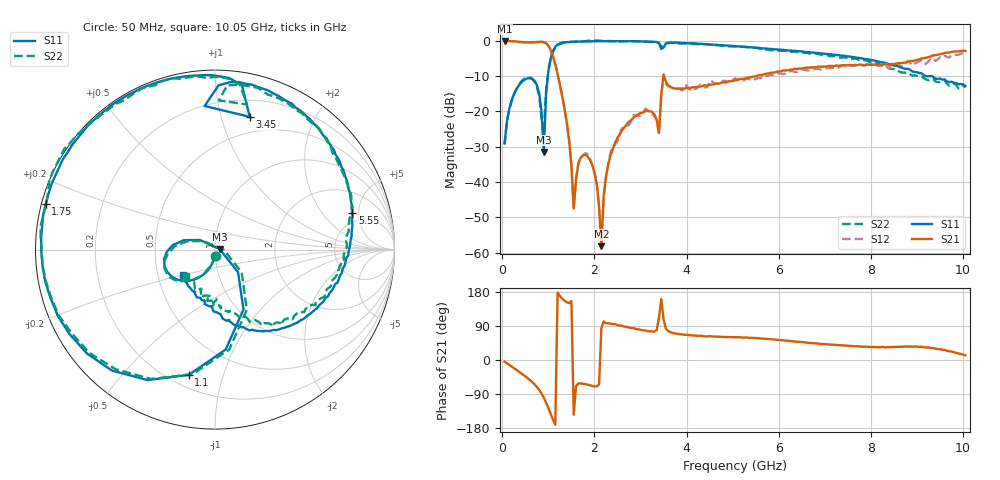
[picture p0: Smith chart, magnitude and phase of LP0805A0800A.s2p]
! AVX THIN FILM OPERATION
! 0805 Size Low Pass Filter P/N  LP0805A0800AWTR
! Network Analyzer HP8720ES.07.64: Feb 23, 2000 Serial No. US39172382
! Hewlett-Packard
!  2 Feb 2003  02:44:22
! Frequency  S11  S21  S12  S22
#	 HZ  S  DB 	R  50
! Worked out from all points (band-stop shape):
!   201 points, 50 MHz to 10.05 GHz, reference 50 ohm
!   highest |S21| = -0.02 dB at 50 MHz (marker M1); lowest = -58.2 dB at 2.15 GHz (marker M2)
!   |S21| within 3 dB of the highest: start of sweep to 1.061 GHz; 9.901 GHz to end of sweep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
!   lowest |S11| = -31.5 dB at 900 MHz (marker M3), VSWR 1.05, Z = 52.7 + j0.312 ohm
!   |S11| at or under -10 dB: start of sweep to 989.2 MHz; 9.188 GHz to 9.278 GHz (90.19 MHz wide, 0.977 % of centre); 9.311 GHz to end of sweep
!   |S22| runs from -29.4 to 0.1 dB; largest |S21 - S12| = 0.14
!   S11 on the Smith chart (normalised r, x): 50 MHz: 0.99, -0.07; 1.1 GHz: 0.27, -0.78; 1.75 GHz: 0.01, +0.13; 3.45 GHz: 0.35, +1.24; 5.55 GHz: 3.81, +4.21; 10.05 GHz: 0.67, -0.20
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5e7  -29.02 -93.7  -0.02 -4.6  -0.00 -4.3  -29.38 -85.1
2.5e8  -15.25 -118.4  -0.17 -21.3  -0.18 -21.6  -15.29 -119.0
6e8  -10.57 -161.9  -0.49 -52.9  -0.43 -52.8  -10.46 -160.5
8e8  -14.82 163.2  -0.32 -78.9  -0.32 -79.2  -15.69 163.8
9e8  -31.54 6.4  -0.39 -99.2  -0.39 -99.0  -26.25 -0.4
9.5e8  -14.91 -44.5  -0.68 -112.3  -0.73 -111.9  -14.14 -40.6
1.1e9  -2.94 -101.8  -4.49 -157.5  -4.97 -156.8  -3.04 -100.1
1.4e9  -0.40 -163.8  -23.23 152.4  -23.50 152.7  -0.43 -164.1
1.55e9  -0.28 -179.4  -47.49 -144.4  -47.36 -138.8  -0.31 -179.5
1.75e9  -0.21 165.0  -32.41 -62.7  -32.71 -63.7  -0.21 164.4
2.05e9  -0.14 146.4  -40.59 -69.6  -40.23 -69.9  0.09 146.3
2.15e9  -0.13 141.1  -58.18 83.8  -57.71 53.8  0.01 141.8
2.25e9  -0.09 135.8  -38.36 96.7  -39.00 95.4  -0.06 136.5
2.5e9  -0.09 123.8  -27.46 91.6  -28.48 93.9  -0.15 124.2
3.1e9  -0.19 97.9  -19.97 78.1  -19.30 77.2  -0.26 97.2
3.4e9  -0.65 80.7  -26.12 111.5  -26.27 110.6  -0.62 81.5
3.45e9  -2.33 75.3  -15.40 160.7  -15.27 157.5  -1.64 77.5
5.05e9  -1.51 31.6  -11.21 60.1  -10.63 57.2  -1.65 28.6
5.55e9  -2.03 15.1  -9.83 57.5  -10.55 54.7  -2.12 14.6
6.75e9  -3.33 -22.5  -7.50 44.1  -8.04 44.5  -3.55 -22.9
8.4e9  -6.72 -69.8  -6.73 33.7  -7.66 29.3  -7.88 -66.0
1.005e10  -12.83 -142.3  -2.91 12.2  -3.81 11.1  -13.21 -137.9
